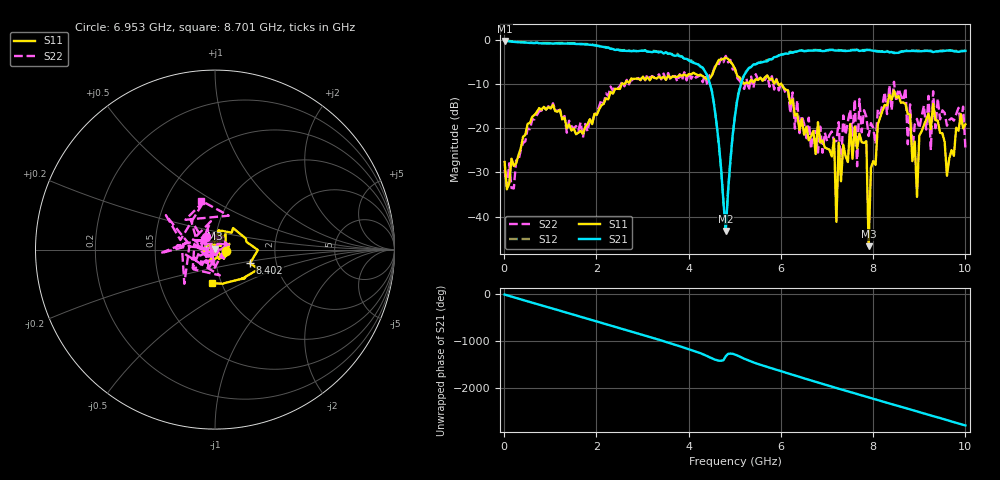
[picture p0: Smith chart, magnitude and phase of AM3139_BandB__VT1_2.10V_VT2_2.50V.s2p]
! Date/Time: Tue, Nov 13, 2018 4:59 PM
! Network Analyzer: Agilent Technologies E8364B Rev: A.07.50.67
! Sweep from 0.010 to 10.000 GHz, 201 Points, Sweep Type: LIN
! Power Supply: 2.101 V, 0.000 A
# Hz S DB R 50
!freq MagS11 AngS11 MagS21 AngS21 MagS12 AngS12 MagS22 AngS22
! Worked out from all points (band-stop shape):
!   201 points, 10 MHz to 10 GHz, reference 50 ohm
!   highest |S21| = -0.27 dB at 10 MHz (marker M1); lowest = -43.2 dB at 4.805 GHz (marker M2)
!   |S21| within 3 dB of the highest: start of sweep to 3.622 GHz; 6.062 GHz to end of sweep
!   lowest |S11| = -46.7 dB at 7.902 GHz (marker M3), VSWR 1.01, Z = 50.1 + j0.445 ohm
!   |S11| at or under -10 dB: start of sweep to 2.552 GHz; 2.594 GHz to 2.611 GHz (16.6 MHz wide, 0.638 % of centre); 6.009 GHz to end of sweep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
!   |S22| runs from -33.6 to -3.7 dB; largest |S21 - S12| = 0.026
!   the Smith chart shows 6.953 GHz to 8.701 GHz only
!   S11 on the Smith chart (normalised r, x): 6.953 GHz: 1.13, -0.02; 8.402 GHz: 1.46, -0.23; 8.701 GHz: 0.90, -0.35
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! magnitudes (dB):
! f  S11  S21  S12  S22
! 10 MHz  -27.6  -0.3  -0.2  -29.4
! 1.708 GHz  -21.2  -1.0  -1.0  -22.2
! 3.357 GHz  -8.4  -2.9  -2.7  -7.8
! 4.406 GHz  -9.0  -8.1  -8.1  -10.4
! 4.805 GHz  -4.1  -43.2  -42.5  -3.7
! 5.005 GHz  -6.6  -17.2  -17.1  -6.7
! 6.703 GHz  -20.6  -2.5  -2.3  -20.7
! 6.953 GHz  -24.4  -2.6  -2.4  -21.0
! 7.153 GHz  -22.5  -2.4  -2.3  -23.0
! 7.203 GHz  -41.2  -2.5  -2.2  -22.9
! 7.253 GHz  -23.3  -2.5  -2.4  -18.6
! 7.852 GHz  -22.9  -2.3  -2.3  -17.4
! 7.902 GHz  -46.7  -2.3  -2.3  -21.8
! 7.952 GHz  -29.0  -2.4  -2.2  -18.9
! 8.352 GHz  -12.4  -2.9  -2.8  -10.3
! 8.402 GHz  -13.6  -2.8  -2.8  -16.0
! 8.701 GHz  -14.6  -2.6  -2.6  -10.9
! 8.951 GHz  -35.5  -2.6  -2.5  -17.9
! 9.251 GHz  -20.2  -2.6  -2.5  -25.0
! 9.301 GHz  -14.5  -2.8  -2.7  -11.7
! 9.6 GHz  -30.7  -2.5  -2.4  -19.5
! 10 GHz  -19.1  -2.6  -2.4  -24.4
